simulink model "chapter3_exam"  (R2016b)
settings: Solver=ode45  StartTime=0.0  StopTime=2.5  RelTol=1e-3  EnableMultiTasking=on
PreLoadFcn:
  | initialize_para;
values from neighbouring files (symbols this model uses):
  delta = 0.25    [initialize_para.m]
  E = 0.7    [initialize_para.m]
  Kt = 0.05    [initialize_para.m]
  N = 100    [initialize_para.m]    (also in main.m = walk_para.N; walk_parameter.m = 5)

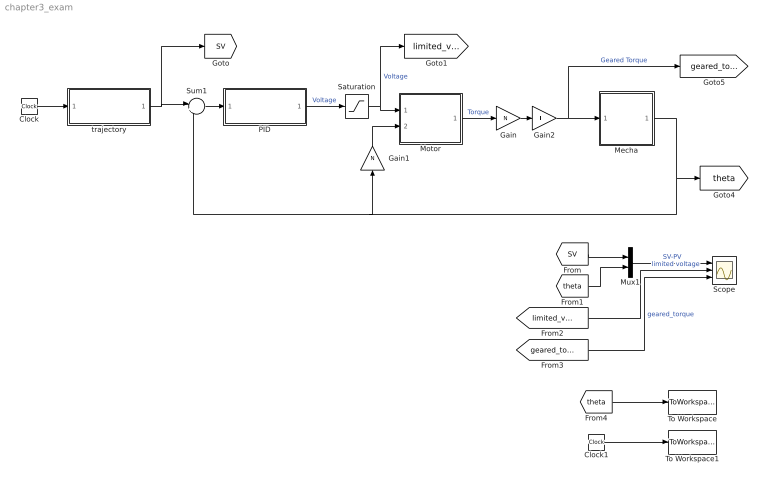
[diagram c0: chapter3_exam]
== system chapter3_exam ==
  Clock : Clock
  Clock1 : Clock
  Gain : Gain  Gain=N
  Gain1 : Gain  Gain=N
  Gain2 : Gain  Gain=E
  Mecha : Subsystem
  Motor : Subsystem
  Mux1 : Mux  Inputs=2
  PID : Subsystem
  Saturation : Saturate
  Scope : Scope  NumInputPorts=3
  Sum1 : Sum  Inputs=|+-
  To Workspace : ToWorkspace  VariableName=theta  SampleTime=0.1
  To Workspace1 : ToWorkspace  VariableName=t  SampleTime=0.1
  trajectory : Subsystem
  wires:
  trajectory/1(theta*(t)) -> Sum1/1, [SV]
  Sum1/1 -> PID/1(Error)
  Mecha/1(Theta) -> Sum1/2, Gain1/1, [theta]
  PID/1(Out1) -> Saturation/1  "Voltage"
  Motor/1(Torque) -> Gain/1  "Torque"
  Clock/1 -> trajectory/1(t)
  Gain1/1 -> Motor/2(theta)
  Gain/1 -> Gain2/1
  Gain2/1 -> [geared_torque], Mecha/1(Torque)  "Geared Torque"
  Saturation/1 -> [limited_voltage], Motor/1(Voltage)  "Voltage"
  [SV] -> Mux1/1
  [theta] -> Mux1/2
  Mux1/1 -> Scope/1  "SV-PV"
  [limited_voltage] -> Scope/2  "limited voltage"
  [geared_torque] -> Scope/3  "geared_torque"
  [theta] -> To Workspace/1
  Clock1/1 -> To Workspace1/1

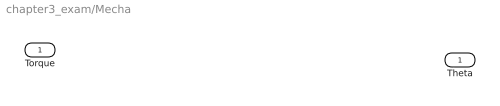
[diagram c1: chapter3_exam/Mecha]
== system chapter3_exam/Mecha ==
  Torque : Inport
  Theta : Outport
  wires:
  ? -> Theta/1

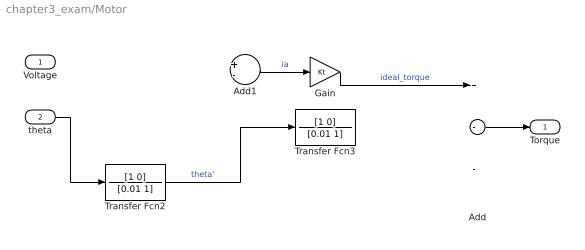
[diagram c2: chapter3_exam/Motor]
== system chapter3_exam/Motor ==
  Voltage : Inport
  theta : Inport  Port=2
  Add : Sum  Inputs=+--
  Add1 : Sum  Inputs=+-
  Gain : Gain  Gain=Kt
  Transfer Fcn2 : TransferFcn  Numerator=[1 0]  Denominator=[0.01 1]
  Transfer Fcn3 : TransferFcn  Numerator=[1 0]  Denominator=[0.01 1]
  Torque : Outport
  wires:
  ? -> Add1/1
  ? -> Add1/2
  Add1/1 -> Gain/1  "ia"
  Voltage/1 -> ?
  Gain/1 -> Add/1  "ideal_torque"
  theta/1 -> Transfer Fcn2/1
  Transfer Fcn3/1 -> ?  "theta''"
  ? -> Add/2
  ? -> Add/3
  Add/1 -> Torque/1
  Transfer Fcn2/1 -> Transfer Fcn3/1  "theta'"

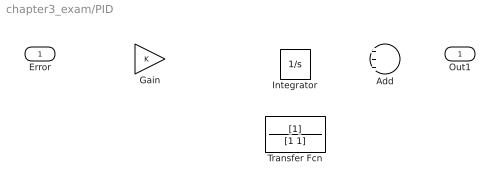
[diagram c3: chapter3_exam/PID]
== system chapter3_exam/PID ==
  Error : Inport
  Add : Sum  Inputs=+++
  Gain : Gain
  Integrator : Integrator
  Transfer Fcn : TransferFcn  Denominator=[1 1]
  Out1 : Outport

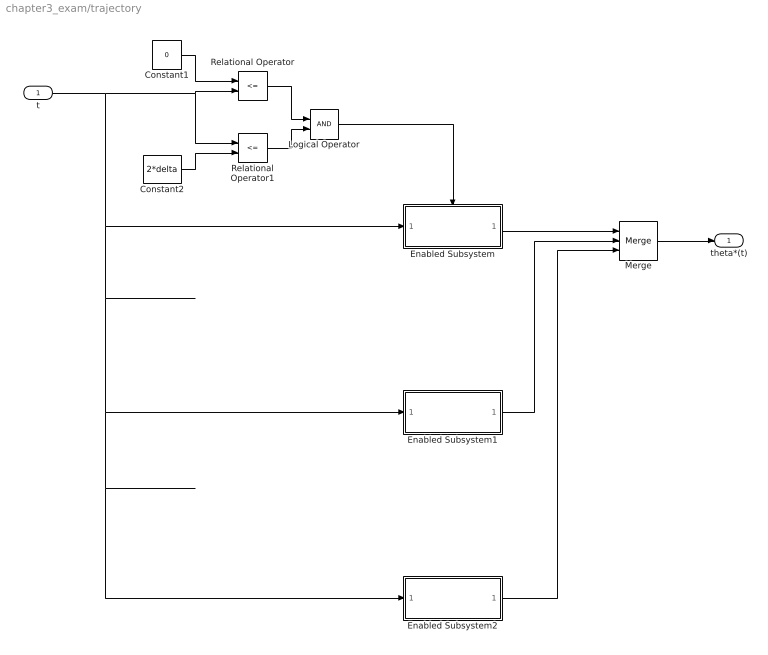
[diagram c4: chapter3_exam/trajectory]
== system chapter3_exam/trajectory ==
  t : Inport
  Constant1 : Constant  Value=0
  Constant2 : Constant  Value=2*delta
  Enabled Subsystem : Subsystem  TreatAsAtomicUnit=on
  Enabled Subsystem1 : Subsystem  TreatAsAtomicUnit=on
  Enabled Subsystem2 : Subsystem  TreatAsAtomicUnit=on
  Logical Operator : Logic  AllPortsSameDT=off  OutDataTypeStr=boolean
  Merge : Merge  Inputs=3
  Relational Operator : RelationalOperator  Operator=<=  OutDataTypeStr=boolean
  Relational Operator1 : RelationalOperator  Operator=<=  OutDataTypeStr=boolean
  theta*(t) : Outport
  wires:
  t/1 -> Relational Operator/2, Relational Operator1/1, Enabled Subsystem/1(t), Enabled Subsystem2/1(t), Enabled Subsystem1/1(t)
  Constant1/1 -> Relational Operator/1
  Relational Operator/1 -> Logical Operator/1
  Constant2/1 -> Relational Operator1/2
  Relational Operator1/1 -> Logical Operator/2
  Logical Operator/1 -> Enabled Subsystem/Enable
  Enabled Subsystem/1(Out1) -> Merge/1
  Merge/1 -> theta*(t)/1
  ? -> ?
  ? -> ?
  ? -> ?
  ? -> ?
  Enabled Subsystem1/1(Out1) -> Merge/2
  ? -> Enabled Subsystem1/Enable
  ? -> ?
  ? -> ?
  ? -> ?
  ? -> ?
  Enabled Subsystem2/1(Out1) -> Merge/3
  ? -> Enabled Subsystem2/Enable

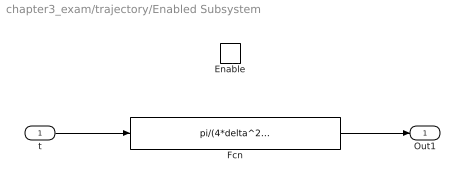
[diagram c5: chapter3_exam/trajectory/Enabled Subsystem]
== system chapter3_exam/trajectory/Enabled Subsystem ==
  t : Inport
  Enable : EnablePort
  Fcn : Fcn  Expr=pi/(4*delta^2)*u[1]^3-pi/(16*delta^3)*u[1]^4
  Out1 : Outport
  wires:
  t/1 -> Fcn/1
  Fcn/1 -> Out1/1

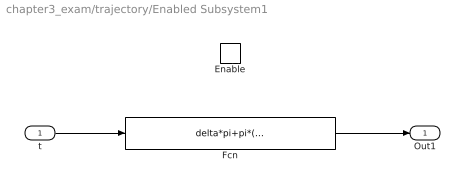
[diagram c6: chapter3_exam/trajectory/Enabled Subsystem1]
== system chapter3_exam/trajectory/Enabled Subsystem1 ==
  t : Inport
  Enable : EnablePort
  Fcn : Fcn  Expr=delta*pi+pi*(u[1]-2*delta)
  Out1 : Outport
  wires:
  Fcn/1 -> Out1/1
  t/1 -> Fcn/1

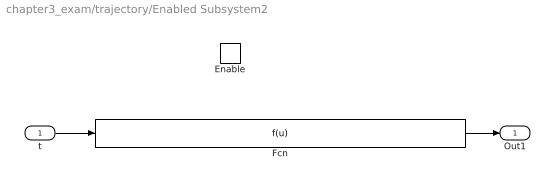
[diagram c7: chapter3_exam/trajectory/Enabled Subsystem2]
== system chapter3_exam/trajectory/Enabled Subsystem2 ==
  t : Inport
  Enable : EnablePort
  Fcn : Fcn
  Out1 : Outport
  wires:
  t/1 -> Fcn/1
  Fcn/1 -> Out1/1
